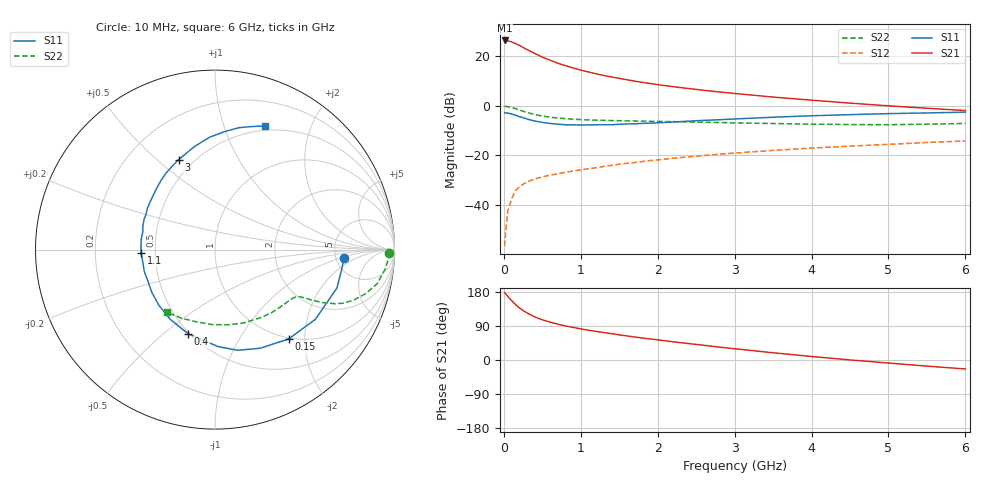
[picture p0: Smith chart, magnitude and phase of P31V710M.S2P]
! SIEMENS Small Signal Semiconductors
! BFP181
! Si NPN RF Bipolar Junction Transistor in SOT143
! VCE = 1.75 V  IC = 10 mA
! Common Emitter S-Parameters:  March  1996
# GHz  S  MA  R  50
!  f  S11  S21  S12  S22
! GHz  MAG  ANG  MAG  ANG  MAG  ANG  MAG  ANG
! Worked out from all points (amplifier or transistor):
!   36 points, 10 MHz to 6 GHz, reference 50 ohm
!   highest |S21| = 26.2 dB at 10 MHz (marker M1)
!   |S21| within 3 dB of that: start of sweep to 261 MHz
!   unconditionally stable (mu >= 1): 877 MHz to end of sweep
!   at 250 MHz: K = 0.40, MSG = 27.5 dB, |S12| = -31.6 dB
!   at 1.4 GHz: K = 1.21, MAG = 15.0 dB, |S12| = -24.0 dB
!   at 6 GHz: K = 1.05, MAG = 4.7 dB, |S12| = -14.2 dB
!   S11 on the Smith chart (normalised r, x): 10 MHz: 5.88, -1.16; 150 MHz: 0.98, -1.67; 400 MHz: 0.49, -0.61; 1.1 GHz: 0.42, -0.02; 3 GHz: 0.42, +0.59; 6 GHz: 0.45, +1.38
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0.01  0.7188 -3.8  20.5 177.5  0.0015 81.7  0.9676 -1.0
0.02  0.7161 -7.5  20.49 175.6  0.0025 77.9  0.9696 -2.4
0.05  0.7122 -17.5  20.25 168.0  0.0075 83.4  0.9562 -6.2
0.1  0.6809 -34.8  19.12 156.9  0.0133 72.3  0.9232 -11.9
0.15  0.645 -50.5  17.81 146.7  0.0195 66.9  0.8733 -16.4
0.2  0.6047 -65.3  16.37 137.8  0.0233 61.3  0.8227 -20.0
0.25  0.5752 -77.3  14.8 130.5  0.0263 57.9  0.7742 -22.7
0.3  0.5406 -88.2  13.53 124.5  0.0293 54.8  0.7327 -24.3
0.4  0.4926 -107.6  11.26 113.9  0.0336 51.2  0.6661 -26.3
0.5  0.4615 -122.7  9.477 106.1  0.037 48.1  0.6196 -27.3
0.6  0.4405 -135.2  8.235 100.0  0.0403 48.0  0.5876 -27.9
0.7  0.4249 -146.1  7.153 94.7  0.0427 47.9  0.5647 -28.4
0.9  0.4125 -163.0  5.739 86.0  0.0488 47.7  0.5362 -29.4
1.1  0.412 -177.1  4.768 78.5  0.0541 48.0  0.5179 -30.9
1.3  0.4151 171.8  4.048 72.4  0.06 48.3  0.5077 -32.9
1.6  0.4295 157.1  3.322 63.6  0.0694 48.3  0.4961 -36.2
2.2  0.4692 134.4  2.411 48.0  0.0878 46.7  0.4775 -44.9
3  0.541 112.0  1.763 29.7  0.1117 42.3  0.4511 -58.6
3.5  0.5867 101.0  1.491 19.1  0.1263 39.0  0.4386 -68.7
4.5  0.661 85.0  1.127 0.1  0.1538 31.5  0.4182 -91.7
5.5  0.7153 73.4  0.888 -16.1  0.1822 24.2  0.425 -115.6
6  0.7426 68.1  0.8 -23.7  0.1956 20.0  0.4405 -127.7
